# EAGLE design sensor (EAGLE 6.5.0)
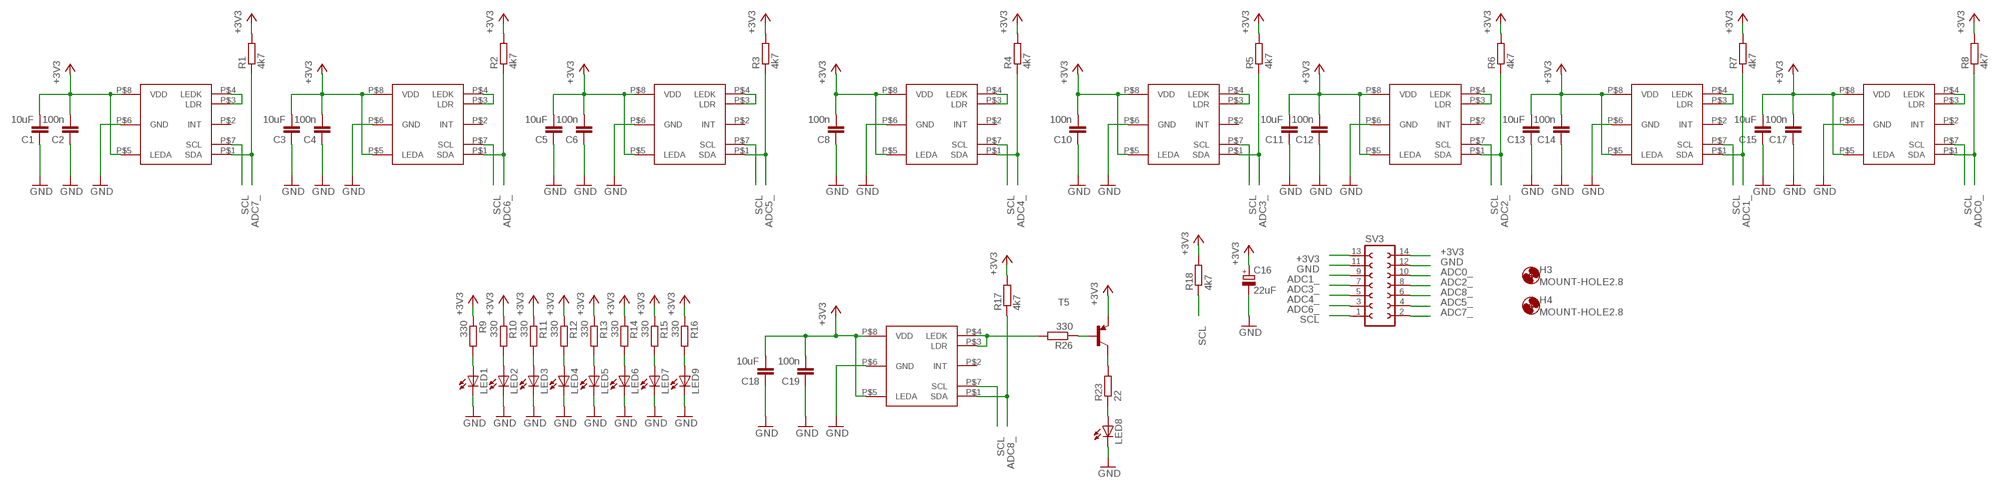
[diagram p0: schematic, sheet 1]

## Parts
C1  10uF  C-EUC0805  [C0805]
C2  100n  C-EUC0805  [C0805]
C3  10uF  C-EUC0805  [C0805]
C4  100n  C-EUC0805  [C0805]
C5  10uF  C-EUC0805  [C0805]
C6  100n  C-EUC0805  [C0805]
C8  100n  C-EUC0805  [C0805]
C10  100n  C-EUC0805  [C0805]
C11  10uF  C-EUC0805  [C0805]
C12  100n  C-EUC0805  [C0805]
C13  10uF  C-EUC0805  [C0805]
C14  100n  C-EUC0805  [C0805]
C15  10uF  C-EUC0805  [C0805]
C16  22uF  CPOL-EU153CLV-0505  [153CLV-0505]
C17  100n  C-EUC0805  [C0805]
C18  10uF  C-EUC0805  [C0805]
C19  100n  C-EUC0805  [C0805]
H3  MOUNT-HOLE2.8  [2,8]
H4  MOUNT-HOLE2.8  [2,8]
LED1  LEDCHIPLED_1206  [CHIPLED_1206]
LED2  LEDCHIPLED_1206  [CHIPLED_1206]
LED3  LEDCHIPLED_1206  [CHIPLED_1206]
LED4  LEDCHIPLED_1206  [CHIPLED_1206]
LED5  LEDCHIPLED_1206  [CHIPLED_1206]
LED6  LEDCHIPLED_1206  [CHIPLED_1206]
LED7  LEDCHIPLED_1206  [CHIPLED_1206]
LED8  LED5MM  [LED5MM]
LED9  LEDCHIPLED_1206  [CHIPLED_1206]
R1  4k7  R-EU_M0805  [M0805]
R2  4k7  R-EU_M0805  [M0805]
R3  4k7  R-EU_M0805  [M0805]
R4  4k7  R-EU_M0805  [M0805]
R5  4k7  R-EU_M0805  [M0805]
R6  4k7  R-EU_M0805  [M0805]
R7  4k7  R-EU_M0805  [M0805]
R8  4k7  R-EU_M0805  [M0805]
R9  330  R-EU_M0805  [M0805]
R10  330  R-EU_M0805  [M0805]
R11  330  R-EU_M0805  [M0805]
R12  330  R-EU_M0805  [M0805]
R13  330  R-EU_M0805  [M0805]
R14  330  R-EU_M0805  [M0805]
R15  330  R-EU_M0805  [M0805]
R16  330  R-EU_M0805  [M0805]
R17  4k7  R-EU_M0805  [M0805]
R18  4k7  R-EU_M0805  [M0805]
R23  22  R-EU_M0805  [M0805]
R26  330  R-EU_M0805  [M0805]
SV3  FE07-2  [FE07-2]
T5  BC857A-PNP-SOT23-BEC  [SOT23-BEC]
U$1  APDS9950  [APDS9950]
U$2  APDS9950_EDGE  [APDS9950_EDGE]
U$4  APDS9950  [APDS9950]
U$5  APDS9950  [APDS9950]
U$6  APDS9950  [APDS9950]
U$7  APDS9950  [APDS9950]
U$8  APDS9950  [APDS9950]
U$9  APDS9950  [APDS9950]
U$10  APDS9950  [APDS9950]

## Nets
+3V3: C1.2 C2.2 C3.2 C4.2 C5.2 C6.2 C8.2 C10.2 C11.2 C12.2 C13.2 C14.2 C15.2 C16.+ C17.2 C18.2 C19.2 R1.2 R2.2 R3.2 R4.2 R5.2 R6.2 R7.2 R8.2 R9.1 R10.1 R11.1 R12.1 R13.1 R14.1 R15.1 R16.1 R17.2 R18.2 SV3.13 SV3.14 T5.E U$1.P$5(LEDA) U$1.P$8(VDD) U$2.P$5(LEDA) U$2.P$8(VDD) U$4.P$5(LEDA) U$4.P$8(VDD) U$5.P$5(LEDA) U$5.P$8(VDD) U$6.P$5(LEDA) U$6.P$8(VDD) U$7.P$5(LEDA) U$7.P$8(VDD) U$8.P$5(LEDA) U$8.P$8(VDD) U$9.P$5(LEDA) U$9.P$8(VDD) U$10.P$5(LEDA) U$10.P$8(VDD)
ADC0_: R8.1 SV3.10 U$10.P$1(SDA)
ADC1_: R7.1 SV3.9 U$9.P$1(SDA)
ADC2_: R6.1 SV3.8 U$8.P$1(SDA)
ADC3_: R5.1 SV3.7 U$7.P$1(SDA)
ADC4_: R4.1 SV3.5 U$6.P$1(SDA)
ADC5_: R3.1 SV3.4 U$5.P$1(SDA)
ADC6_: R2.1 SV3.3 U$4.P$1(SDA)
ADC7_: R1.1 SV3.2 U$1.P$1(SDA)
ADC8_: R17.1 SV3.6 U$2.P$1(SDA)
GND: C1.1 C2.1 C3.1 C4.1 C5.1 C6.1 C8.1 C10.1 C11.1 C12.1 C13.1 C14.1 C15.1 C16.- C17.1 C18.1 C19.1 LED1.C LED2.C LED3.C LED4.C LED5.C LED6.C LED7.C LED8.K(C) LED9.C SV3.11 SV3.12 U$1.P$6(GND) U$2.P$6(GND) U$4.P$6(GND) U$5.P$6(GND) U$6.P$6(GND) U$7.P$6(GND) U$8.P$6(GND) U$9.P$6(GND) U$10.P$6(GND)
N$1: R23.2 T5.C
N$2: U$4.P$3(LDR) U$4.P$4(LEDK)
N$3: LED1.A R9.2
N$4: U$1.P$3(LDR) U$1.P$4(LEDK)
N$5: LED2.A R10.2
N$6: LED3.A R11.2
N$7: LED4.A R12.2
N$8: LED5.A R13.2
N$9: U$5.P$3(LDR) U$5.P$4(LEDK)
N$13: LED6.A R14.2
N$14: LED7.A R15.2
N$15: U$6.P$3(LDR) U$6.P$4(LEDK)
N$16: LED9.A R16.2
N$19: R26.2 U$2.P$3(LDR) U$2.P$4(LEDK)
N$20: U$7.P$3(LDR) U$7.P$4(LEDK)
N$24: U$8.P$3(LDR) U$8.P$4(LEDK)
N$27: U$9.P$3(LDR) U$9.P$4(LEDK)
N$28: LED8.A R23.1
N$31: U$10.P$3(LDR) U$10.P$4(LEDK)
N$32: R26.1 T5.B
SCL: R18.1 SV3.1 U$1.P$7(SCL) U$2.P$7(SCL) U$4.P$7(SCL) U$5.P$7(SCL) U$6.P$7(SCL) U$7.P$7(SCL) U$8.P$7(SCL) U$9.P$7(SCL) U$10.P$7(SCL)
Unconnected: U$1.P$2(INT) U$2.P$2(INT) U$4.P$2(INT) U$5.P$2(INT) U$6.P$2(INT) U$7.P$2(INT) U$8.P$2(INT) U$9.P$2(INT) U$10.P$2(INT)

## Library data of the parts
C1-C6 C8 C10-C15 C17-C19 = resistor:C-EU: CAPACITOR, European symbol
C16 = resistor:CPOL-EU: POLARIZED CAPACITOR, European symbol
H3 H4 = holes:MOUNT-HOLE: MOUNTING HOLE with drill center marker
LED1-LED7 LED9 = my_parts:LED: LED
LED8 = led:LED: LED
R1-R18 R23 R26 = resistor:R-EU_: RESISTOR, European symbol
SV3 = con-lsta:FE07-2: FEMALE HEADER; OC_FARNELL: unknown; OC_NEWARK: unknown
T5 = transistor:*-PNP-: PNP Transistror
U$1 U$4-U$10 = my_parts:APDS9950
U$2 = my_parts:APDS9950_EDGE

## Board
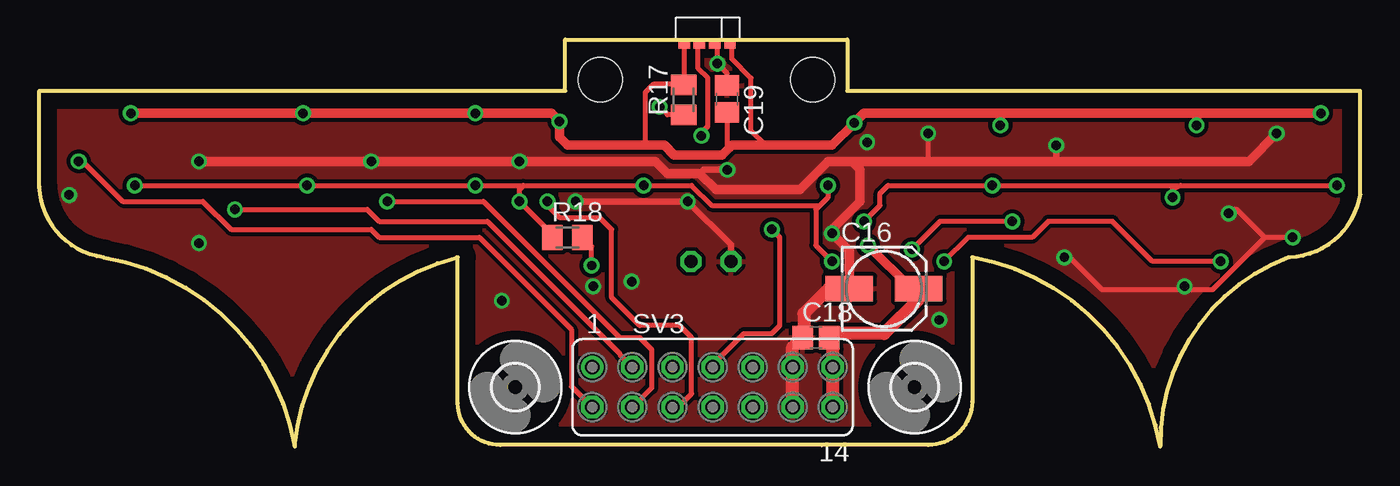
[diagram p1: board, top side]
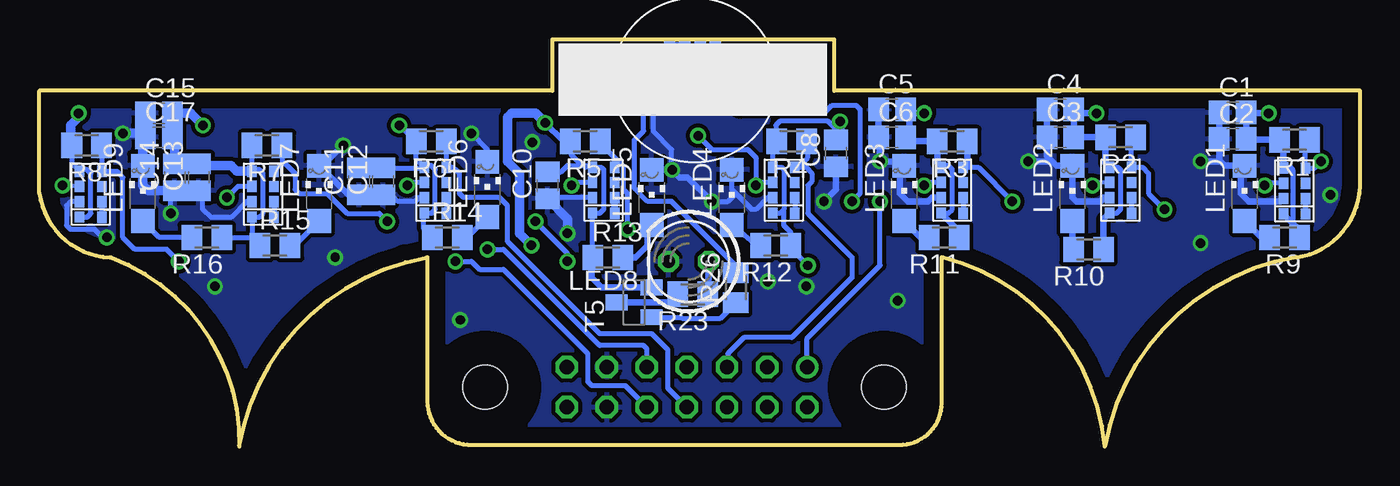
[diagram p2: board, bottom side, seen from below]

Size 83.72 x 25.81 mm. Coordinates in mm from the lower left corner, seen from the top.
Outline: 0,22.55 33.33,22.55 33.33,25.81 51.21,25.81 51.21,22.55 83.72,22.55 83.72,16.05 arc-80 79.25,11.99 79.17,11.99 arc71 71.04,0 arc71 59.16,11.99 59.13,11.99 59.13,2.84 arc-90 56.34,0.1 29.21,0.1 arc-90 26.52,2.74 26.52,11.99 26.47,11.99 arc71 16.18,0 arc71 4.06,11.99 arc-80 0,16.46 0,22.55
Copper layers (1*16): Top 0.035mm / dielectric 1.5mm / Bottom 0.035mm
Design rules "default *": minimum track width 10mil, minimum drill 24mil, track to track 10mil, track to pad 10mil, pad to pad 10mil, via to via 10mil, smd to smd 10mil, copper to edge 40mil, drill to drill 8mil, minimum pad ring 10mil, minimum via ring 8mil, stop-mask expansion 4mil, vias tented up to drill 0mil, thermal gap 10mil

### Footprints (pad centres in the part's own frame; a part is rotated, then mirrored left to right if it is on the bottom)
C0805 = smd 1.3 x 1.5: 1 -0.85,0; 2 0.85,0
153CLV-0505 = smd 3 x 1.6: + 2.2,0; - -2.2,0
2,8 = hole 2.8: 0,0
CHIPLED_1206 = smd 1.5 x 1.5: A 0,-1.75; C 0,1.75
LED5MM = drill 0.813 octagon: A -1.27,0; K 1.27,0
M0805 = smd 1.3 x 1.6: 1 -0.95,0; 2 0.95,0
FE07-2 = drill 0.914: 1 -7.62,1.27 | drill 0.914 octagon: 2 -7.62,-1.27; 3 -5.08,1.27; 4 -5.08,-1.27; 5 -2.54,1.27; 6 -2.54,-1.27; 7 0,1.27; 8 0,-1.27; 9 2.54,1.27; 10 2.54,-1.27; 11 5.08,1.27; 12 5.08,-1.27; 13 7.62,1.27; 14 7.62,-1.27
SOT23-BEC = smd 1 x 1.4: B -0.95,-1.1; C 0,1.1; E 0.95,-1.1
APDS9950 = smd 0.6 x 0.72: P$1 0.7,1.4; P$2 0.7,0.43; P$3 0.7,-0.54; P$4 0.7,-1.51; P$5 -0.7,-1.5; P$6 -0.7,-0.53; P$7 -0.7,0.44; P$8 -0.7,1.41
APDS9950_EDGE = smd 0.6 x 0.72 bottom: P$1 -0.9,1.5; P$2 -0.9,0.53; P$3 -0.9,-0.44; P$4 -0.9,-1.41 | smd 0.6 x 0.72: P$5 -0.9,-1.41; P$6 -0.9,-0.44; P$7 -0.9,0.53; P$8 -0.9,1.5
BALL_3/8 = hole 2.8: -6.35,0; 7.112,0

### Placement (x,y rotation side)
C1  8.08,21.18 0 bottom
C2  8.08,19.51 0 bottom
C3  19,19.61 0 bottom
C4  19,21.39 0 bottom
C5  29.67,21.39 0 bottom
C6  29.67,19.61 0 bottom
C8  33.22,18.59 90 bottom
C10  51.51,16.56 90 bottom
C11  63.45,16.81 90 bottom
C12  61.93,16.81 90 bottom
C13  73.61,17.07 90 bottom
C14  75.13,17.07 90 bottom
C15  76.15,21.13 0 bottom
C16  53.54,10.01 0 top
C17  76.15,19.61 0 bottom
C18  49.23,6.91 0 top
C19  43.59,22.05 270 top
H3  30.18,3.76 0 top
H4  55.47,3.76 0 top
LED1  7.32,16.05 0 bottom
LED2  18.24,16.05 0 bottom
LED3  28.91,16.05 0 bottom
LED4  39.83,15.8 0 bottom
LED5  44.91,15.8 0 bottom
LED6  55.32,16.31 0 bottom
LED7  65.99,16.05 0 bottom
LED8  42.57,11.73 180 bottom
LED9  77.17,16.05 0 bottom
R1  4.17,19.46 180 bottom
R2  15.19,19.61 180 bottom
R3  25.86,19.35 180 bottom
R4  36.02,19.35 180 bottom
R5  49.12,19.35 180 bottom
R6  58.88,19.35 180 bottom
R7  69.29,19.1 180 bottom
R8  80.72,19.1 180 bottom
R9  4.78,13.26 180 bottom
R10  17.22,12.5 180 bottom
R11  26.37,13.26 180 bottom
R12  37.03,12.75 180 bottom
R13  47.7,11.99 0 bottom
R14  57.86,13.26 0 bottom
R15  68.78,12.75 0 bottom
R16  73.1,13.26 180 bottom
R17  40.84,22 90 top
R18  33.48,13.26 0 top
R23  42.32,9.65 180 bottom
R26  39.57,10.06 90 bottom
SV3  42.67,3.76 0 top
T5  46.02,9.14 90 bottom
U$1  4.17,16.26 0 bottom
U$2  42.37,26.42 90 top
U$3  [BALL_3/8]  42.67,23.27 0 bottom
U$4  15.19,16.31 0 bottom
U$5  25.86,16.31 0 bottom
U$6  36.53,16.31 0 bottom
U$7  47.96,16.31 0 bottom
U$8  58.62,16.31 0 bottom
U$9  69.55,16.05 0 bottom
U$10  80.47,16.05 0 bottom

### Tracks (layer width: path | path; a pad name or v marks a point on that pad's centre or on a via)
+3V3  (via drill 0.6)
  Top 0.305: 55.58,9.84 55.58,9.53 55.74,9.36 | v35,11.48 35,12.68 R18.2 | U$2.P$8 40.87,22.97 | C19.2 43.59,19.1 43.74,18.95 | 40.87,22.97 38.92,22.97 38.41,22.45 38.41,19.41 38.71,19.1 | 50.24,19.1 46.03,19.1 45.11,20.01 45.11,23.37 43.89,24.59 43.89,25.4 U$2.P$5 | 40.87,22.97 R17.2
  Top 0.61: v5.79,21.13 v16.71,21.13 v27.64,21.13 32.46,21.13 v32.97,20.62 32.97,19.61 33.48,19.1 38.71,19.1 39.62,19.1 40.23,18.49 43.28,18.49 43.74,18.95 43.89,19.1 50.24,19.1 v51.66,20.52 52.27,21.13 60.91,21.13 | 60.91,21.13 73.36,21.13 | 73.36,21.13 v81.23,21.13 | v60.91,20.37 60.91,21.13 | v73.36,20.37 73.36,21.13 | C16.+ 55.27,10.01 v52.53,12.75
  Top 0.813: SV3.14 SV3.13 50.29,6.69 C18.2 50.33,7.16 53.54,7.16 55.74,9.36 | 55.58,9.84 C16.+
  Bottom 0.305: U$5.P$5 26.09,14.81 25.86,15.04 25.86,17.58 26.11,17.83 26.44,17.83 U$5.P$8 | U$1.P$8 4.36,17.67 4.27,17.58 4.27,14.16 4.07,13.96 | U$4.P$8 15.33,17.72 15.19,17.58 15.19,15.04 15.44,14.78 15.87,14.78 U$4.P$5 | 36.53,15.04 36.53,17.58 36.67,17.72 U$6.P$8 37.23,19.1 R4.2 37.03,19.42 37.03,20.37 36.78,20.62 33.73,20.62 33.22,20.12 C8.2 | 36.53,15.04 36.78,14.78 37.2,14.78 U$6.P$5 | 36.53,15.04 36.53,14.02 36.08,13.58 R12.1 36.08,12.56 v35,11.48 | U$8.P$8 59.21,17.83 58.88,17.83 58.62,17.58 58.62,15.04 58.85,14.81 U$8.P$5 59.39,14.74 59.39,13.83 R14.1 58.62,12.75 | U$8.P$8 59.83,18.22 R6.2 | U$8.P$8 59.38,17.66 C12.2 C11.2 | U$7.P$8 48.1,17.72 47.96,17.58 47.96,15.04 48.21,14.78 48.63,14.78 U$7.P$5 R13.1 | U$7.P$8 49.11,17.72 49.23,17.83 | C10.2 50.66,17.41 50.24,17.83 49.33,17.83 | 49.23,17.83 48.77,17.83 U$7.P$8 | R7.2 U$9.P$8 70.13,17.58 69.8,17.58 69.55,17.32 69.55,14.78 69.78,14.55 U$9.P$5 70.25,13.26 R15.1 70.24,13.26 R16.1 | C15.2 75.3,20.62 C17.2 | U$10.P$5 80.7,14.55 80.47,14.78 80.47,17.32 80.72,17.58 81.05,17.58 U$10.P$8 81.67,17.97 R8.2 | 49.23,17.83 49.33,17.83 | 49.33,17.83 49.99,18.49 49.99,19.57 R5.2 50.5,19.35
  Bottom 0.406: U$1.P$8 4.87,19.46 R1.2 7.18,19.46 C2.2 | 7.02,19.71 C2.2 | 4.84,14.78 U$1.P$5 4.07,13.96 3.83,13.72 R9.1 | C1.2 C2.2 | U$4.P$8 16.14,17.97 R2.2 C3.2 C4.2 17.9,21.13 v16.71,21.13 | R10.1 16.27,14.42 U$4.P$5 | C2.2 7.23,20.97 7.06,21.13 v5.79,21.13 | 28.56,21.13 28.56,19.86 C6.2 28.56,19.35 R3.2 26.81,17.97 U$5.P$8 | v27.64,21.13 28.56,21.13 | 28.56,21.13 C5.2 | R11.1 25.42,13.66 U$5.P$5 | 50.5,19.35 v51.66,20.52 | T5.E 48.09,10.09 48.72,10.72 48.72,11.92 R13.1 | v60.91,20.37 60.84,20.37 R6.2
  Bottom 0.61: v81.23,21.13 81.23,20.88 81.74,20.37 81.74,19.17 R8.2 | R6.2 59.89,19.35 | C15.2 74.12,21.13 v73.36,20.37 | 75.3,20.62 75.13,20.46 C14.2 C13.2 72.76,17.83 71.58,17.83 71.21,17.46 U$9.P$8 | v52.53,12.75 53.29,13.51 53.29,17.32 54.05,18.08 54.05,20.88 53.8,21.13 52.27,21.13 v51.66,20.52 | v32.97,20.62 32.97,19.7 C8.2
ADC0_  (via drill 0.6)
  Top 0.305: v74.88,11.73 70.56,11.73 68.02,14.27 63.96,14.27 62.94,13.26 58.88,13.26 v57.35,11.73
  Bottom 0.305: R8.1 U$10.P$1 78.82,17.45 78.44,17.07 78.44,13.26 77.67,12.5 75.64,12.5 v74.88,11.73 | v57.35,11.73 56.34,11.73 55.83,11.23 54.31,11.23 48.97,5.89 48.97,4.11 48.72,3.86 46.58,3.86 SV3.10
ADC1_  (via drill 0.6)
  Top 0.305: v61.67,14.27 57.1,14.27 v55.32,12.5
  Bottom 0.305: R7.1 68.34,17.96 | 68.34,17.96 U$9.P$1 | 68.34,17.96 68.15,17.96 67.51,17.32 67.51,16.31 67.26,16.05 65.48,16.05 64.21,14.78 62.18,14.78 v61.67,14.27 | SV3.9 45.21,6.2 45.42,6.4 48.21,6.4 54.31,12.5 v55.32,12.5
ADC2_
  Bottom 0.305: U$8.P$1 R6.1 | U$8.P$1 57.48,17.71 | SV3.8 43.89,3.71 43.89,6.15 44.91,7.16 48.21,7.16 54.05,13 54.05,15.29 54.56,15.8 56.85,15.8 57.1,16.05 57.1,17.32 57.35,17.58 57.79,17.58 U$8.P$1
ADC3_  (via drill 0.6)
  Top 0.305: SV3.7 42.67,5.18 44.65,7.16 46.43,7.16 46.94,7.67 46.94,13.26 v46.43,13.77
  Bottom 0.305: 47.26,18.34 U$7.P$1 47.13,17.83 | v46.43,13.77 46.43,16.05 46.69,16.31 46.69,17.77 47.26,18.34 | R5.1 48.17,19.26 47.26,18.34
ADC4_
  Bottom 0.305: R4.1 35,19.29 35,18.34 35.63,17.71 U$6.P$1 35.13,17.71 34.75,17.32 34.75,16.81 35,16.56 35,14.78 32.21,11.99 32.21,10.72 36.02,6.91 39.07,6.91 40.08,5.89 40.08,5.08 SV3.5
ADC5_  (via drill 0.6)
  Top 0.305: SV3.4 38.81,3.71 38.81,6.15 38.05,6.91 36.78,6.91 28.14,15.54 v22.05,15.54
  Bottom 0.305: 24.91,17.96 U$5.P$1 24.21,17.71 v22.05,15.54
  Bottom 0.406: R3.1 24.91,17.96
ADC6_  (via drill 0.6)
  Top 0.305: v12.4,15.04 20.78,15.04 21.54,14.27 28.4,14.27 36.78,5.89 36.78,5.84 SV3.3
  Bottom 0.305: R2.1 14.49,19.36 U$4.P$1 13.8,17.71 13.41,17.32 13.41,16.05 v12.4,15.04
ADC7_  (via drill 0.6)
  Top 0.305: v2.49,18.08 2.74,18.08 5.28,15.54 10.36,15.54 12.14,13.77 21.03,13.77 21.54,13.26 27.89,13.26 33.73,7.42 33.73,3.81 SV3.2
  Bottom 0.305: R1.1 3.47,19.46 U$1.P$1 2.92,17.66 v2.49,18.08
ADC8_  (via drill 0.6)
  Top 0.305: SV3.6 40.49,2.49 41.35,3.35 41.35,6.91 40.59,7.67 38.05,7.67 36.27,9.45 36.27,13.77 35.51,14.53 32.97,14.53 32.21,15.29 v32.21,15.54 | R17.1 39.81,21.05 v39.32,21.54
  Bottom 0.254: U$2.P$1 40.87,24.31
  Bottom 0.305: v32.21,15.54 31.7,16.05 31.7,21.39 31.95,21.64 33.48,21.64 33.88,21.23 39.01,21.23 v39.32,21.54 39.32,22.76 40.87,24.31
GND  (via drill 0.6)
  Top 0.305: v79.45,13.26 77.67,13.26 | 77.67,13.26 75.9,15.04 75.64,15.04 v75.39,14.78 | v56.34,19.86 56.34,18.08 | v64.97,11.99 65.33,11.99 67.36,9.96 74.37,9.96 77.67,13.26 | U$2.P$6 42.98,25.35 v42.98,24.28 43.59,23.67 C19.1
  Top 0.406: v33.99,15.54 v41.1,15.54 43.84,12.8 LED8.K | v64.47,19.1 64.47,18.08 | v43.61,17.55 42.09,17.55 41.86,17.32
  Top 0.61: v10.11,18.08 v21.03,18.08 v30.43,18.08 39.07,18.08 39.83,17.32 41.86,17.32 42.88,16.31 48.21,16.31 49.99,18.08 51.51,18.08 | v78.44,19.86 76.66,18.08 64.47,18.08 56.34,18.08 51.51,18.08 | C16.- 51.34,12.41 v50.24,13.51 50.24,13.77 52.02,15.54 52.02,17.58 51.51,18.08
  Top 0.813: SV3.12 SV3.11 47.75,6.29 C18.1 48.46,7 48.46,8.43 50.04,10.01 C16.- 51,9.67
  Bottom 0.305: v41.1,15.54 40.08,15.54 39.57,16.05 | C11.1 C12.1 61.23,15.78 61,15.54 59.89,15.54 59.66,15.78 U$8.P$6 | 39.57,16.05 39.83,16.31 LED4.C 39.83,17.83 | U$7.P$6 51.7,15.78 C10.1 | U$9.P$6 70.58,15.52 71.58,14.53 72.85,14.53 73.36,15.04 73.36,15.96 C13.1 | U$10.P$6 81.76,15.52 81.99,15.29 81.99,14.02 81.74,13.77 80.21,13.77 79.71,13.26 v79.45,13.26 | v75.39,14.78 75.39,15.96 C14.1 | LED6.C 55.32,18.85 v56.34,19.86 | 39.57,16.05 38.56,15.04 38.3,15.04 37.56,15.78 U$6.P$6 | 43.64,17.58 43.64,18.85 44.81,20.01 44.81,23.37 44.5,23.67 43.89,23.67 43.28,24.28 v42.98,24.28
  Bottom 0.406: C1.1 C2.1 8.93,18.17 | 8.93,18.17 8.59,17.83 7.34,17.83 LED1.C 7.57,17.55 7.57,16.05 7.06,15.54 5.05,15.54 U$1.P$6 | C4.1 C3.1 19.85,18.43 19.51,18.08 | 19.51,18.08 19.25,17.83 18.27,17.83 LED2.C 18.24,15.8 17.98,15.54 16.46,15.54 16.23,15.78 U$4.P$6 | v21.03,18.08 19.51,18.08 | v10.11,18.08 9.02,18.08 8.93,18.17 | C5.1 C6.1 30.43,19.52 v30.43,18.08 29.19,18.08 LED3.C 29.16,17.55 29.16,16.05 28.65,15.54 27.38,15.54 27.15,15.78 U$5.P$6 | 32.88,18.08 C8.1 33.22,16.31 v33.99,15.54 | v64.47,19.1 65.76,17.8 LED7.C 64.15,15.96 C11.1 | LED5.C v43.61,17.55 | v43.61,17.55 43.13,17.07 42.62,17.07 v41.1,15.54 | v43.61,17.55 43.64,17.58
  Bottom 0.61: 77,20.12 C17.1 77.17,19.44 LED9.C 77.17,16.56 76.82,16.22 C14.1 C13.1 | 77,20.12 C15.1 | v78.44,19.86 77.25,19.86 77,20.12 | v50.24,13.51 50.24,14.44 C10.1
  other vias: 10.11,12.9 1.88,15.95 29.31,9.25 37.54,10.46 35.1,10.16 57.05,8.03 52.48,19.3 72.59,10.16
  pour Top: -5.49,33.12 85.04,33.12 85.04,-4.67 -5.49,-4.67
  pour Bottom: -6.1,30.68 86.87,30.68 86.87,-9.25 -6.1,-9.25
N$1
  Bottom 0.406: T5.C 43.77,9.14 R23.2
N$2
  Bottom 0.305: U$4.P$3 U$4.P$4
N$3
  Bottom 0.406: R9.2 6.27,13.26 LED1.A
N$4
  Bottom 0.305: U$1.P$3 U$1.P$4
N$5
  Bottom 0.406: LED2.A 18.24,12.56 R10.2
N$6
  Bottom 0.406: R11.2 27.86,13.26 LED3.A
N$7
  Bottom 0.305: R12.2 38.28,12.75 LED4.A
N$8
  Bottom 0.406: R13.2 45.92,11.99 45.16,12.75 45.16,13.79 LED5.A
N$9
  Bottom 0.305: U$5.P$3 U$5.P$4
N$13
  Bottom 0.305: R14.2 56.62,13.26 LED6.A
N$14
  Bottom 0.305: R15.2 67.54,12.75 LED7.A
N$15
  Bottom 0.305: U$6.P$3 U$6.P$4
N$16
  Bottom 0.305: R16.2 76.12,13.26 LED9.A
N$19
  Bottom 0.305: R26.2 39.27,11.18 43.64,15.54 45.16,15.54 46.03,16.41 46.03,19.41 45.42,20.01 45.42,23.88 U$2.P$4 U$2.P$3
N$20
  Bottom 0.406: U$7.P$3 U$7.P$4
N$24
  Bottom 0.305: U$8.P$3 U$8.P$4
N$27
  Bottom 0.305: U$9.P$3 U$9.P$4
N$28
  Bottom 0.406: LED8.A 41.3,9.72 R23.1
N$31
  Bottom 0.305: U$10.P$3 U$10.P$4
N$32
  Bottom 0.305: T5.B 43.04,8.19 42.98,8.13 40.55,8.13 R26.1
SCL  (via drill 0.6)
  Top 0.305: v27.64,16.56 27.38,16.56 | v6.05,16.56 v16.97,16.56 v27.64,16.56 | 30.68,16.56 30.43,16.31 v30.43,15.54 32.02,13.95 R18.1 | v27.64,16.56 30.68,16.56 | 30.68,16.56 v38.3,16.56 41.35,16.56 42.62,15.29 49.48,15.29 | 72.34,16.56 v60.4,16.56 53.8,16.56 53.29,16.05 53.29,15.29 v52.27,14.27 | 72.34,16.56 v82.25,16.56 | v71.83,15.8 71.83,16.31 72.34,16.56 | 49.48,15.29 49.99,15.8 v49.99,16.56 | 49.48,15.29 49.23,15.04 49.23,12.75 v50.24,11.73 | v41.96,19.71 41.96,19.91 42.37,20.32 42.37,23.37 41.76,23.98 41.76,25.44 U$2.P$7
  Bottom 0.254: U$4.P$7 16.78,16.75 v16.97,16.56 | v82.25,16.56 81.24,16.56 U$10.P$7
  Bottom 0.305: U$1.P$7 5.91,16.7 v6.05,16.56 | U$5.P$7 27.45,16.75 v27.64,16.56 | SV3.1 35.05,6.86 30.43,11.48 v30.43,15.54 | U$6.P$7 38.12,16.75 v38.3,16.56 38.3,18.34 38.81,18.85 41.1,18.85 v41.96,19.71 | U$9.P$7 71.14,16.49 v71.83,15.8 | U$8.P$7 60.22,16.75 v60.4,16.56 | U$7.P$7 49.8,16.75 v49.99,16.56 | v50.24,11.73 50.24,12.24 v52.27,14.27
